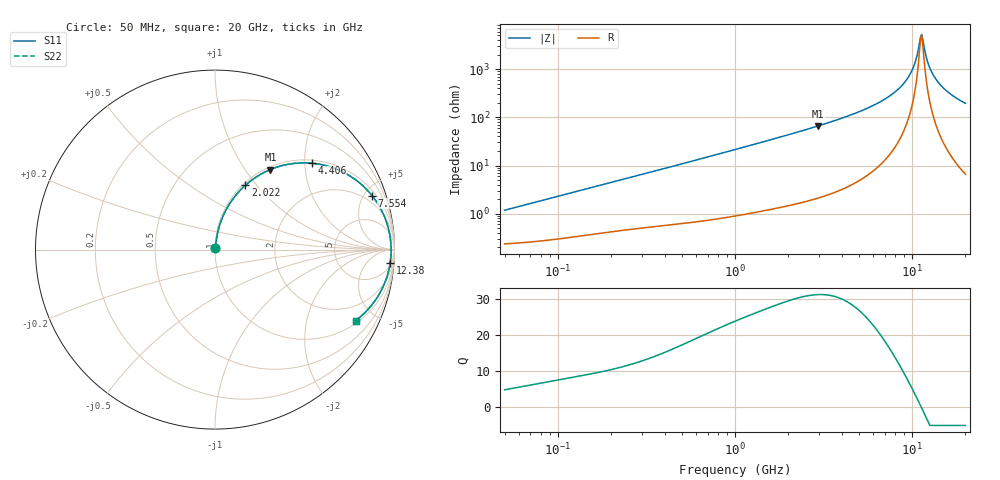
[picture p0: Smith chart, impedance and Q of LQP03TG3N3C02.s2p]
!Murata Part Number: LQP03TG3N3C02
!These Parameters are Measured in Series Mode Connection
!  o--[Z]--o
!Port1  Port2
!  o-------o
!Freq. Start=50[MHz] Stop=20[GHz], 401[Steps]
# Hz S RI R 50
!Freq.(Hz) S11(Real) S11(Imag) S21(Real) S21(Imag) S12(Real) S12(Imag) S22(Real) S22(Imag)
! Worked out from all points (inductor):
!   401 points, 50 MHz to 20 GHz, reference 50 ohm
!   read as one part in series: L = 3.67 nH near 51.52 MHz
!   highest Q = 31.3 at 2.94 GHz (marker M1), where L = 3.57 nH
!   self-resonance near 11.15 GHz
!   S11 on the Smith chart (normalised r, x): 50 MHz: 1.00, +0.02; 2.022 GHz: 1.03, +0.88; 4.406 GHz: 1.07, +2.17; 7.554 GHz: 1.36, +5.67; 12.38 GHz: 7, -24; 20 GHz: 1.13, -3.89
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5e7  0.00249 0.0115  0.9975 -0.0115  0.9975 -0.0115  0.00249 0.0115
1.364002e8  0.00441 0.0305  0.9956 -0.0305  0.9956 -0.0305  0.00441 0.0305
3.721004e8  0.0119 0.0793  0.9881 -0.0793  0.9881 -0.0793  0.0119 0.0793
1e9  0.0515 0.2011  0.9485 -0.2011  0.9485 -0.2011  0.0515 0.2011
2.021818e9  0.1695 0.3588  0.8305 -0.3588  0.8305 -0.3588  0.1695 0.3588
2.728004e9  0.2751 0.4308  0.7249 -0.4308  0.7249 -0.4308  0.2751 0.4308
2.940159e9  0.3087 0.4463  0.6913 -0.4463  0.6913 -0.4463  0.3087 0.4463
4.405649e9  0.5386 0.4816  0.4614 -0.4816  0.4614 -0.4816  0.5386 0.4816
5.944466e9  0.7366 0.4194  0.2634 -0.4194  0.2634 -0.4194  0.7366 0.4194
7.442007e9  0.8676 0.3099  0.1324 -0.3099  0.1324 -0.3099  0.8676 0.3099
7.554318e9  0.8751 0.3008  0.1249 -0.3008  0.1249 -0.3008  0.8751 0.3008
8.774992e9  0.9374 0.1992  0.0626 -0.1992  0.0626 -0.1992  0.9374 0.1992
9.745021e9  0.9658 0.1192  0.0342 -0.1192  0.0342 -0.1192  0.9658 0.1192
1.034674e10  0.9756 0.0713  0.0244 -0.0713  0.0244 -0.0713  0.9756 0.0713
1.115139e10  0.9811 0.0103  0.0189 -0.0103  0.0189 -0.0103  0.9811 0.0103
1.131968e10  0.9813 -0.00194  0.0187 0.00194  0.0187 0.00194  0.9813 -0.00194
1.149051e10  0.9811 -0.0142  0.0189 0.0142  0.0189 0.0142  0.9811 -0.0142
1.238412e10  0.9758 -0.0753  0.0242 0.0753  0.0242 0.0753  0.9758 -0.0753
1.334722e10  0.963 -0.1351  0.037 0.1351  0.037 0.1351  0.963 -0.1351
1.482269e10  0.9328 -0.2148  0.0672 0.2148  0.0672 0.2148  0.9328 -0.2148
1.696185e10  0.8755 -0.3062  0.1245 0.3062  0.1245 0.3062  0.8755 -0.3062
2e10  0.7833 -0.3953  0.2167 0.3953  0.2167 0.3953  0.7833 -0.3953
